(* Logix 5000 AddOnInstructionDefinition export AMCI_3204_AOP_Hold; software revision 20.03 *)

ADD_ON_INSTRUCTION AMCI_3204_AOP_Hold   (* revision 1.0, vendor AMCI, ExecuteEnableInFalse *)
VAR_INPUT
   channel_number : INT; {required}
END_VAR
VAR_IN_OUT
   AMCI_3204_output_data : AM:1756_3204:O:0; {required}
END_VAR
VAR
   command_data_block : DINT[8]; {access None}
END_VAR

ROUTINE EnableInFalse   (* ladder *)
END_ROUTINE

ROUTINE Logic   (* ladder *)
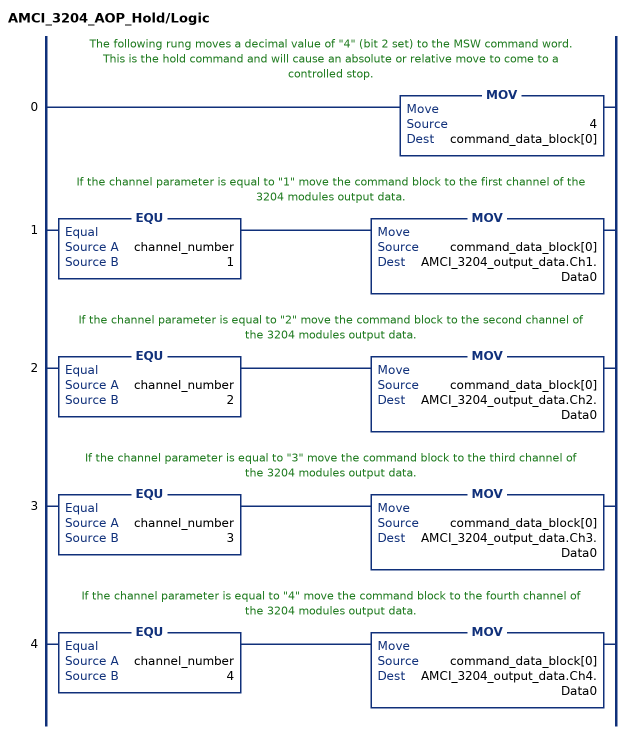
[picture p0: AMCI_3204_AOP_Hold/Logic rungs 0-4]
   // The following rung moves a decimal value of "4" (bit 2 set) to the MSW command word.  This is the hold command and will cause an absolute or relative move to come to a controlled stop.
   0: MOV(4,command_data_block[0]);
   // If the channel parameter is equal to "1" move the command block to the first channel of the 3204 modules output data.
   1: EQU(channel_number,1)MOV(command_data_block[0],AMCI_3204_output_data.Ch1.Data0);
   // If the channel parameter is equal to "2" move the command block to the second channel of the 3204 modules output data.
   2: EQU(channel_number,2)MOV(command_data_block[0],AMCI_3204_output_data.Ch2.Data0);
   // If the channel parameter is equal to "3" move the command block to the third channel of the 3204 modules output data.
   3: EQU(channel_number,3)MOV(command_data_block[0],AMCI_3204_output_data.Ch3.Data0);
   // If the channel parameter is equal to "4" move the command block to the fourth channel of the 3204 modules output data.
   4: EQU(channel_number,4)MOV(command_data_block[0],AMCI_3204_output_data.Ch4.Data0);
END_ROUTINE
END_ADD_ON_INSTRUCTION
